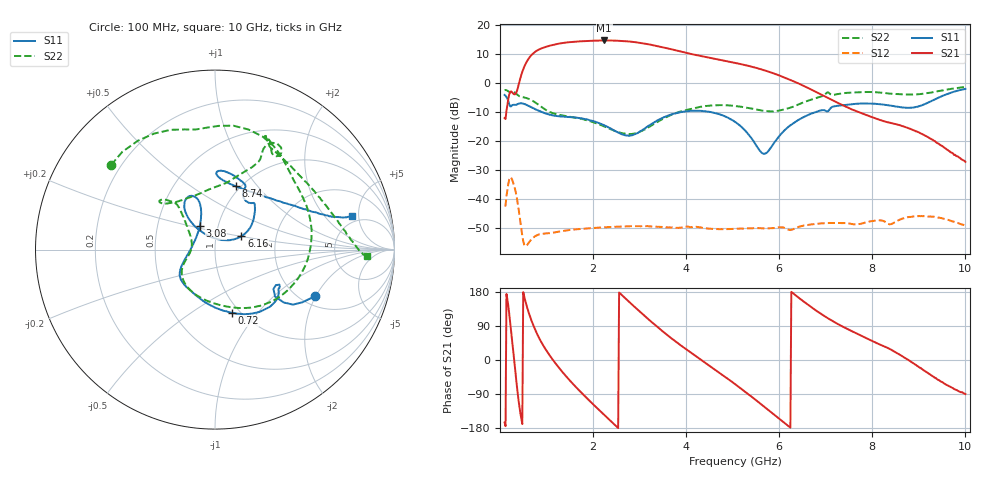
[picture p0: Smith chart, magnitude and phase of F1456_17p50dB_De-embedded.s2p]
! Integrated Device Technology
! Corporate Headquarters
! 6024 Silver Creek Valley Road
! San Jose, CA 95138  USA
! Phone:  1-408-284-8200
! Toll Free:  1-800-223-1366
! Webpage:  http://www.idt.com/
! Timing and RF Division
! 515 Groton Road, Suite 102
! Westford, MA 01886-6024
! Device:  F1456
! Description: 6-bit 0.5 dB Transmit Variable Gain Amplifier
! Frequency:  2100.0 -  2950.00 MHz
! Package:  6x6 mm Thin QFN Plastic Package: 28 pin
! State:  35
! Atten State:  17.5 dB
! Voltage:  +5.00 Volts
! Current:  216.983 mA
! Data:  The device was measured on a the F1455 evaluation board which has
!  individual transmission lines to the RF pins.  Data was collected
!  using a calibrated network analyzer.  The evaluation board was
!  de-embedded using a TRL calibration technique.
!  The reference plane is the edge of the package pin.
!  Pin  1 = CSb
!  Pin  2 = DATA
!  Pin  3 = CLK
!  Pin  4 = RSET
!  Pin  5 = GND
!  Pin  6 = RFIN  = Port 1
!  Pin  7 = GND
!  Pin  8 = NC
!  Pin  9 = NC
!  Pin 10 = NC
!  Pin 11 = NC
!  Pin 12 = NC
!  Pin 13 = NC
!  Pin 14 = /STBY
!  Pin 15 = GND
!  Pin 16 = RFOUT  = Port 2
!  Pin 17 = GND
!  Pin 18 = NC
!  Pin 19 = NC
!  Pin 20 = NC
!  Pin 21 = GND
!  Pin 22 = NC
!  Pin 23 = GND
!  Pin 24 = NC
!  Pin 25 = NC
!  Pin 26 = NC
!  Pin 27 = GND
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# GHz S dB R 50
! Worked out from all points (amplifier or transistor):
!   496 points, 100 MHz to 10 GHz, reference 50 ohm
!   highest |S21| = 14.6 dB at 2.24 GHz (marker M1)
!   |S21| within 3 dB of that: 853.4 MHz to 3.673 GHz (2.82 GHz wide, 125 % of centre)
!   unconditionally stable (mu >= 1): start of sweep to end of sweep
!   at 1.74 GHz: K = 28.06, MAG = 14.8 dB, |S12| = -50.3 dB
!   at 5.06 GHz: K = 59.76, MAG = 7.8 dB, |S12| = -50.3 dB
!   at 10 GHz: K = 361.80, MAG = -17.6 dB, |S12| = -49.1 dB
!   S11 on the Smith chart (normalised r, x): 100 MHz: 2.36, -1.99; 720 MHz: 0.91, -0.74; 3.08 GHz: 0.82, +0.22; 6.16 GHz: 1.33, +0.20; 8.74 GHz: 0.95, +0.78; 10 GHz: 4.20, +4.06
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0.1  -4.19 -25.0  -12.17 -165.1  -42.29 48.6  -2.54 140.8
0.24  -8.12 -30.3  -2.97 74.0  -32.67 -74.4  -3.34 94.3
0.32  -7.61 -31.3  -4.00 -17.0  -36.39 -149.9  -3.31 67.2
0.44  -7.07 -41.2  1.70 -141.4  -48.11 136.2  -4.76 38.0
0.56  -7.54 -56.9  6.81 149.0  -56.26 155.0  -5.19 11.8
0.72  -8.77 -75.4  10.20 90.6  -53.25 140.9  -6.41 -23.5
0.96  -10.46 -99.7  12.22 32.3  -51.93 97.0  -9.09 -67.9
1.18  -11.36 -116.9  13.19 -6.7  -51.52 72.7  -10.68 -95.9
1.48  -11.78 -133.4  13.95 -51.2  -50.74 48.7  -11.62 -123.4
1.76  -12.27 -144.0  14.30 -87.6  -50.28 31.4  -12.47 -140.1
2.24  -14.65 -159.6  14.57 -144.9  -49.75 6.6  -15.02 -159.3
2.62  -17.75 173.8  14.41 171.2  -49.50 -11.6  -17.37 -176.8
3.08  -16.06 122.6  13.57 119.4  -49.40 -33.7  -16.28 152.6
3.4  -12.82 109.8  12.58 85.4  -49.57 -48.5  -13.36 138.2
4.1  -9.67 114.1  9.93 19.8  -49.72 -78.5  -9.02 131.6
5.06  -13.56 130.8  6.83 -64.4  -50.26 -122.3  -8.00 139.3
5.66  -24.43 81.2  4.40 -121.5  -50.14 -156.7  -9.63 122.4
6.16  -15.66 27.1  1.45 -170.8  -50.34 171.6  -8.92 86.0
6.7  -10.56 42.0  -2.43 138.4  -48.73 146.3  -5.74 65.1
8.36  -7.79 87.7  -13.68 30.1  -48.70 73.8  -3.72 62.3
8.74  -8.60 71.7  -15.40 2.4  -46.33 66.3  -4.04 49.0
10  -2.12 13.8  -27.23 -89.9  -49.13 -21.4  -1.46 -2.6
